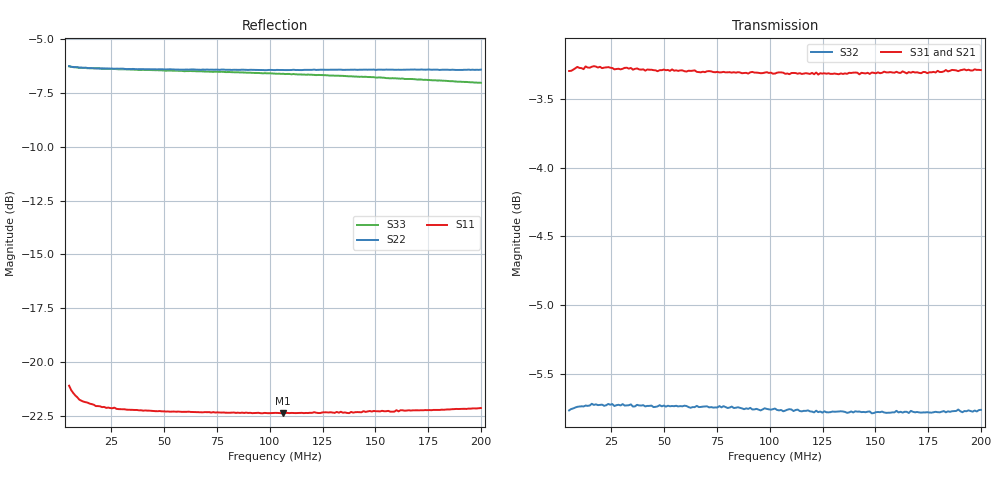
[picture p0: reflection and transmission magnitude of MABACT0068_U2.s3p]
#	MHz	S	RI	R	75
!FREQ	R1	I1	R2	I2	R3	I3
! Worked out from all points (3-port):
!   201 points, 5 MHz to 200 MHz, reference 75 ohm
!   strongest paths, dB at 5 MHz, 53.75 MHz, 102.5 MHz, 151.2 MHz, 200 MHz:
!     S31: -3.3, -3.3, -3.3, -3.3, -3.3
!     S21: -3.3, -3.3, -3.4, -3.5, -3.5
!     S32: -5.8, -5.7, -5.8, -5.8, -5.8
!   lowest |S11| = -22.4 dB at 106.4 MHz (marker M1), VSWR 1.17, Z = 64.5 + j1.81 ohm
!   |S11| at or under -10 dB: start of sweep to end of sweep
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5  -0.0859 0.0206  0.6836 0.0065  -0.6841 -0.00668
   0.6839 0.00665  -0.4852 0.0155  -0.5121 -0.00574
   -0.6841 -0.00668  -0.5149 -0.00653  -0.4847 0.0158
6.95  -0.0833 0.0166  0.6851 0.00101  -0.6849 -6.1e-05
      0.6849 0.00061  -0.483 0.0146  -0.5137 -0.00208
      -0.6849 -6.1e-05  -0.5157 -0.00125  -0.4826 0.0151
9.875  -0.0809 0.0133  0.686 -0.00613  -0.6859 0.00708
       0.687 -0.00589  -0.4815 0.0149  -0.5147 0.00259
       -0.6859 0.00708  -0.5165 0.00278  -0.4808 0.0159
17.675  -0.0786 0.0102  0.6859 -0.0193  -0.6863 0.0211
        0.6868 -0.0193  -0.4795 0.0179  -0.5149 0.012
        -0.6863 0.0211  -0.5174 0.0115  -0.4795 0.0192
22.55  -0.0779 0.0094  0.686 -0.0268  -0.6856 0.0285
       0.6862 -0.0265  -0.4789 0.0199  -0.5144 0.0163
       -0.6856 0.0285  -0.5169 0.0158  -0.4781 0.022
52.775  -0.0763 0.00952  0.6811 -0.0668  -0.6805 0.0706
        0.6813 -0.0672  -0.4758 0.0387  -0.5124 0.0422
        -0.6805 0.0706  -0.5149 0.043  -0.472 0.0429
102.5  -0.0752 0.0138  0.6659 -0.1299  -0.6687 0.1371
       0.6656 -0.1311  -0.4698 0.0722  -0.5057 0.0829
       -0.6687 0.1371  -0.5088 0.0842  -0.4599 0.0771
106.4  -0.075 0.014  0.6638 -0.1343  -0.6682 0.1419
       0.6645 -0.1347  -0.4697 0.0746  -0.5047 0.0862
       -0.6682 0.1419  -0.5071 0.0868  -0.4593 0.0799
154.175  -0.0746 0.0194  0.6444 -0.1905  -0.653 0.2026
         0.6432 -0.1914  -0.4641 0.1065  -0.4967 0.1234
         -0.653 0.2026  -0.499 0.1233  -0.443 0.1094
200  -0.0738 0.0266  0.618 -0.2432  -0.6337 0.2592
     0.6182 -0.2445  -0.4556 0.1396  -0.4871 0.1591
     -0.6337 0.2592  -0.4898 0.1597  -0.4229 0.1362
